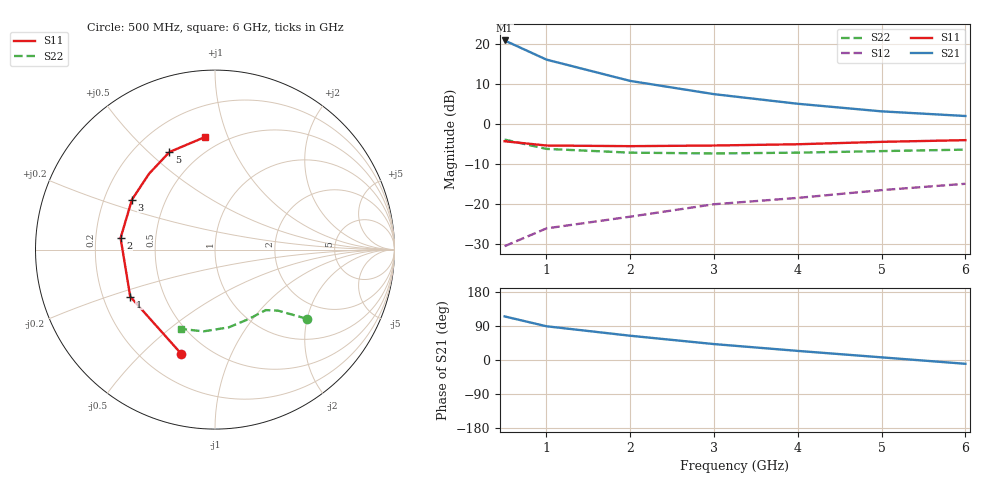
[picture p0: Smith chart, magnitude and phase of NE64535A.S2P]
! FILENAME:  NE64535A.S2P  VERSION: 1.0
! NEC PART NUMBER: NE64535  DATE:  8/79
! BIAS CONDITIONS: VCE=8V, IC=7MA
# GHZ S MA R 50
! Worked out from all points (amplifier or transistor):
!   7 points, 500 MHz to 6 GHz, reference 50 ohm
!   highest |S21| = 20.9 dB at 500 MHz (marker M1)
!   |S21| within 3 dB of that: start of sweep to 813.7 MHz
!   unconditionally stable (mu >= 1): 1.705 GHz to 5.266 GHz
!   at 1 GHz: K = 0.79, MSG = 21.0 dB, |S12| = -26.0 dB
!   at 3 GHz: K = 1.11, MAG = 11.7 dB, |S12| = -20.0 dB
!   at 6 GHz: K = 0.91, MSG = 8.5 dB, |S12| = -14.9 dB
!   lowest NFmin = 0.90 dB at 500 MHz
!   S11 on the Smith chart (normalised r, x): 500 MHz: 0.36, -0.66; 1 GHz: 0.32, -0.23; 2 GHz: 0.31, +0.06; 3 GHz: 0.32, +0.25; 5 GHz: 0.34, +0.58; 6 GHz: 0.40, +0.83
0.5  0.61 -108.0  11.03 115.0  0.03 37.0  0.64 -37.0
1  0.54 -151.0  6.36 89.0  0.05 39.0  0.49 -44.0
2  0.53 173.0  3.45 64.0  0.07 43.0  0.44 -50.0
3  0.54 149.0  2.36 42.0  0.1 44.0  0.43 -64.0
4  0.56 131.0  1.79 24.0  0.12 43.0  0.44 -80.0
5  0.6 115.0  1.44 7.0  0.15 39.0  0.46 -98.0
6  0.63 95.0  1.26 -10.0  0.18 33.0  0.48 -113.0
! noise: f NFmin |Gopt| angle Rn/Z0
0.5  0.9  0.19  71  0.23
1  1.1  0.23  73  0.19
1.5  1.5  0.24  148  0.1
2  1.9  0.41  176  0.06
2.5  2.1  0.36  -161  0.09
3  2.7  0.45  -150  0.13
3.5  2.9  0.37  -149  0.22
4  3.4  0.53  -129  0.36
